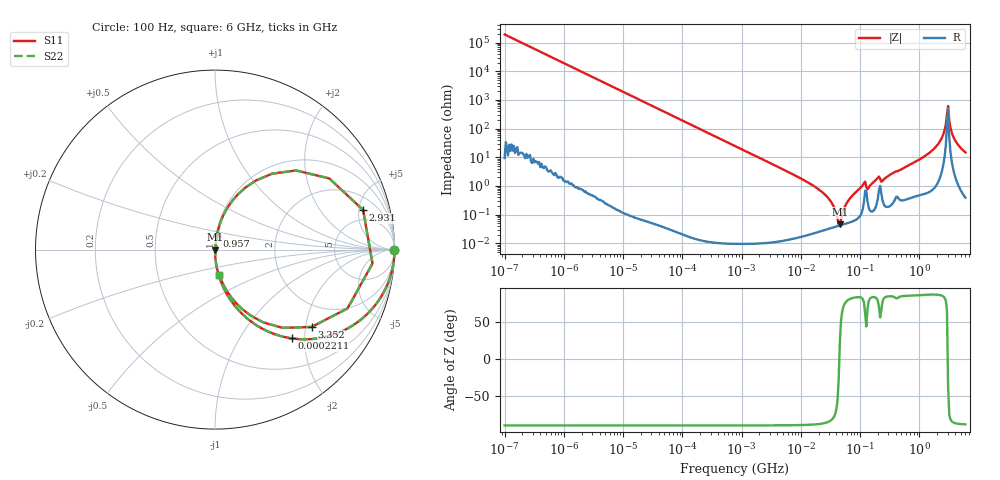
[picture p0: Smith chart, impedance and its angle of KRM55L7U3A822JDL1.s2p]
!Murata Part Number: KRM55L7U3A822JDL1
!These Parameters are Measured in Series Mode Connection
!Data Generated on Jan 08, 2026
!  o--ll--o
!Port1  Port2
!  o------o
!Operation Temp=25[degC], DC Bias Voltage=0[V]
!Freq. Start=100[Hz] Stop=6[GHz] 401[Steps]
# Hz S RI R 50
!Freq.(Hz) S11(Real) S11(Imag) S21(Real) S21(Imag) S12(Real) S12(Imag) S22(Real) S22(Imag)
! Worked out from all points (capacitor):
!   401 points, 100 Hz to 6 GHz, reference 50 ohm
!   read as one part in series: C = 8.33 nF near 109 Hz
!   lowest |Z| = 45.1 mohm at 45.56 MHz (marker M1)
!   series resonance near 44.69 MHz, so ESL is about 1.5 nH
!   S11 on the Smith chart (normalised r, x): 100 Hz: open; 221.1 kHz: 1.00, -1.73; 957 MHz: 1.01, +0.16; 2.931 GHz: 3.42, +5.58; 3.352 GHz: 1.32, -2.16; 6 GHz: 1.01, -0.30
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100  1 -0.000524  3e-07 0.000524  3e-07 0.000524  1 -0.000524
2008  0.9999 -0.0105  0.000111 0.0105  0.000111 0.0105  0.9999 -0.0105
40335  0.9573 -0.2022  0.0427 0.2022  0.0427 0.2022  0.9573 -0.2022
94437  0.8035 -0.3973  0.1965 0.3973  0.1965 0.3973  0.8035 -0.3973
221108  0.4274 -0.4946  0.5726 0.4946  0.5726 0.4946  0.4274 -0.4946
774597  0.0574 -0.2323  0.9426 0.2323  0.9426 0.2323  0.0574 -0.2323
1.555665e7  0.000326 -0.0107  0.9997 0.0107  0.9997 0.0107  0.000326 -0.0107
2.911731e7  0.000332 -0.00372  0.9997 0.00372  0.9997 0.00372  0.000332 -0.00372
4.556224e7  0.00042 0.000165  0.9996 -0.000165  0.9996 -0.000165  0.00042 0.000165
6.233367e7  0.000514 0.00287  0.9995 -0.00287  0.9995 -0.00287  0.000514 0.00287
1.115611e8  0.00173 0.0106  0.9983 -0.0106  0.9983 -0.0106  0.00173 0.0106
1.395531e8  0.00184 0.00855  0.9982 -0.00855  0.9982 -0.00855  0.00184 0.00855
1.909225e8  0.0026 0.0169  0.9974 -0.0169  0.9974 -0.0169  0.0026 0.0169
2.497637e8  0.0026 0.0162  0.9974 -0.0162  0.9974 -0.0162  0.0026 0.0162
3.124326e8  0.00247 0.0233  0.9975 -0.0233  0.9975 -0.0233  0.00247 0.0233
9.569533e8  0.0106 0.0772  0.9894 -0.0772  0.9894 -0.0772  0.0106 0.0772
2.142435e9  0.1011 0.2777  0.8989 -0.2777  0.8989 -0.2777  0.1011 0.2777
2.562649e9  0.317 0.4226  0.683 -0.4226  0.683 -0.4226  0.317 0.4226
2.931063e9  0.8254 0.2203  0.1746 -0.2203  0.1746 -0.2203  0.8254 0.2203
3.352442e9  0.5384 -0.4308  0.4616 0.4308  0.4616 0.4308  0.5384 -0.4308
4.009986e9  0.1457 -0.3264  0.8543 0.3264  0.8543 0.3264  0.1457 -0.3264
6e9  0.0249 -0.1434  0.9751 0.1434  0.9751 0.1434  0.0249 -0.1434
